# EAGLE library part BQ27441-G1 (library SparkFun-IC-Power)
Texas Instruments BQ27441-G1 LiPo Battery Fuel Gauge The Texas Instruments bq27441-G1 fuel gauge is a microcontroller peripheral that provides system-side fuel gauging for single-cell Li-Ion batteries. The device requires minimal user configuration and system microcontroller firmware development. The bq27441-G1 battery fuel gauge uses the patented Impedance Track™ algorithm for fuel gauging, and provides information such as remaining battery capacity (mAh), state-of-charge (%), and battery voltage (mV). Datasheet SparkFun Products SparkFun Battery Babysitter (PRT-13777)
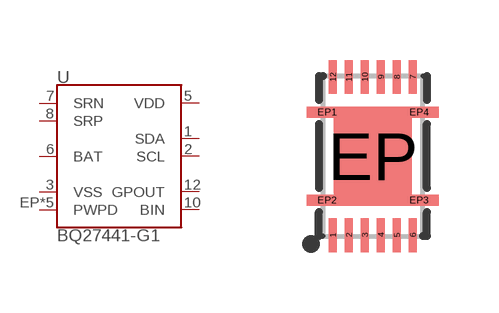
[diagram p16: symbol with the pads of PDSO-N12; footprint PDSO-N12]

Designator prefix U

## BQ27441-G1 (PROD_ID: IC-13220)  [PDSO-N12]
1  SDA
2  SCL
3  VSS
5  VDD
6  BAT
7  SRN
8  SRP
10  BIN
12  GPOUT
EP  PWPD
EP1  PWPD
EP2  PWPD
EP3  PWPD
EP4  PWPD

## Footprint PDSO-N12 (pad centres in mm)
12-Pin VSON 2.5 x 4.0 mm IC Dimensions: 2.5 x 4.0 x 1.0 mm Pitch: 0.4mm Pins: 12 + Bottom Pad Used by the BQ27441 LiPo Fuel Gauge Example Datasheet
smd 0.2 x 0.85: 1 -1,-1.975; 2 -0.6,-1.975; 3 -0.2,-1.975; 4 0.2,-1.975; 5 0.6,-1.975; 6 1,-1.975; 7 1,1.975; 8 0.6,1.975; 9 0.2,1.975; 10 -0.2,1.975; 11 -0.6,1.975; 12 -1,1.975
smd 1.95 x 1.95: EP 0,0
smd 1 x 0.25: EP1 -1.15,1.1; EP2 -1.15,-1.1; EP3 1.15,-1.1; EP4 1.15,1.1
